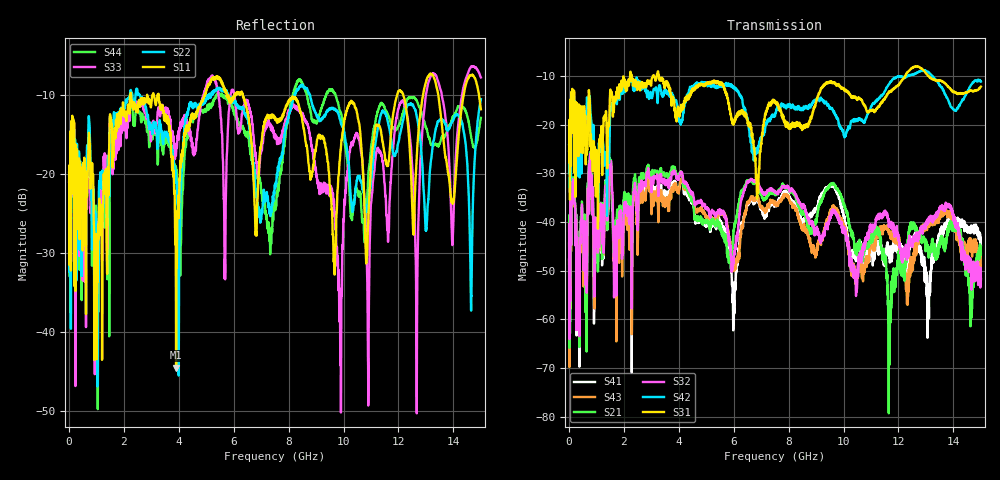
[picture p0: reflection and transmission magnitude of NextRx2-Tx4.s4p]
! FILE: N:\QM 2007\Prüfprotokolle\Highspeed\Konfektionierte Ltg\L45593-D106\D30\8216\0002\Next\NextRx2-Tx4.s4p
# MHz S DB R 50.00
! FREQ  S11  S12  S13  S14
!  S21  S22  S23  S24
!  S31  S32  S33  S34
!  S41  S42  S43  S44
!  DB  ANG  DB  ANG  DB  ANG  DB  ANG
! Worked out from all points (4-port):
!   2999 points, 10 MHz to 15 GHz, reference 50 ohm
!   strongest paths, dB at 10 MHz, 3.755 GHz, 7.505 GHz, 11.26 GHz, 15 GHz:
!     S31: -25.3, -14.6, -15.2, -16.3, -12.2
!     S42: -24.2, -13.5, -18.3, -14.9, -11.2
!     S32: -40.5, -30.0, -33.8, -38.7, -51.8
!     S21: -47.9, -28.7, -34.4, -41.8, -46.4
!     S43: -44.5, -33.3, -36.2, -42.7, -51.9
!     S41: -47.7, -32.3, -36.7, -44.3, -44.8
!   lowest |S11| = -44.5 dB at 3.905 GHz (marker M1), VSWR 1.01, Z = 50.3 + j0.515 ohm
!   |S11| at or under -10 dB: start of sweep to 2.247 GHz; 3.27 GHz to 4.955 GHz (1.685 GHz wide, 41 % of centre); 6.334 GHz to 11.95 GHz (5.613 GHz wide, 61.4 % of centre)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
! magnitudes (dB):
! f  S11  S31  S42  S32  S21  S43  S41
! 10 MHz  -19.8  -25.3  -24.2  -40.5  -47.9  -44.5  -47.7
! 3.905 GHz  -44.5  -17.9  -15.0  -30.7  -30.4  -32.6  -32.5
! 6.005 GHz  -10.4  -19.3  -12.5  -47.6  -41.9  -48.6  -61.2
! 9.875 GHz  -17.8  -12.2  -20.3  -40.1  -34.5  -39.5  -36.0
! 11.67 GHz  -17.4  -13.3  -11.6  -40.0  -69.4  -42.4  -47.4
! 14.64 GHz  -7.5  -13.1  -11.9  -48.7  -56.8  -45.2  -40.9
! 15 GHz  -11.8  -12.2  -11.2  -51.8  -46.4  -51.9  -44.8
